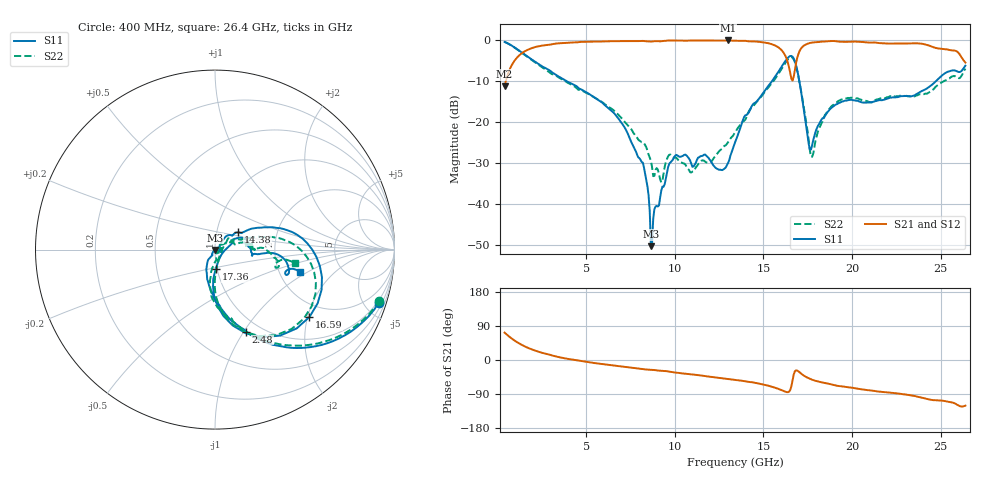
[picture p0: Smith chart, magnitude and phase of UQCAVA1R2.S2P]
!  Part Number  UQCAVA1R2 	Mounting Orientation: Horizontal
!  Description: Ultra Low ESR Microwave capacitors
!  Application: Coupling, Bypass, Tuning, DC Block
!  Filters, Matching
# GHZ S DB R 50
! Freq  |S11|  S11 Ph  |S21|  S21 Ph  |S12|  S12 Ph  |S22|  S22 Ph
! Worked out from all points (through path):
!   401 points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, 400 MHz to 26.4 GHz, reference 50 ohm
!   highest |S21| = 0.00 dB at 13.01 GHz (marker M1); lowest = -11.2 dB at 400 MHz (marker M2)
!   group delay of S21, straight-line fit = 15 ps
!   lowest |S11| = -50.3 dB at 8.655 GHz (marker M3), VSWR 1.01, Z = 49.9 - j0.268 ohm
!   |S11| at or under -10 dB: 3.914 GHz to 15.48 GHz (11.57 GHz wide, 119 % of centre); 17.03 GHz to 24.72 GHz (7.69 GHz wide, 36.8 % of centre)
!   |S22| runs from -34.7 to -0.4 dB; largest |S21 - S12| = 0.0052
!   S11 on the Smith chart (normalised r, x): 400 MHz: 0.83, -6.19; 2.48 GHz: 0.85, -1.02; 14.38 GHz: 1.27, +0.25; 16.59 GHz: 1.59, -2.06; 17.36 GHz: 0.99, -0.22; 26.4 GHz: 2.60, -0.86
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0.4  -0.36 -18.0  -11.17 72.1  -11.20 72.1  -0.37 -17.3
1.18  -2.37 -45.5  -3.83 44.8  -3.85 44.9  -2.40 -44.1
2.48  -6.23 -69.2  -1.29 19.4  -1.31 19.5  -6.46 -70.4
4.755  -12.04 -92.9  -0.35 -3.1  -0.36 -3.0  -12.23 -94.3
7.225  -21.68 -121.0  -0.17 -18.4  -0.16 -18.2  -20.15 -97.3
8.265  -31.10 -125.4  -0.15 -24.5  -0.13 -24.2  -25.11 -79.7
8.655  -50.30 -118.5  -0.26 -25.9  -0.24 -25.6  -29.46 -76.2
9.11  -40.35 1.2  -0.21 -27.9  -0.19 -27.7  -32.67 -37.7
10.085  -27.98 3.5  -0.01 -33.4  -0.01 -33.2  -28.67 5.9
10.995  -30.89 -13.9  -0.01 -37.9  -0.01 -37.8  -32.08 33.7
13.01  -29.93 35.5  0.00 -50.2  -0.01 -50.2  -24.92 33.2
13.4  -24.95 49.0  -0.07 -52.6  -0.05 -52.5  -22.50 29.9
14.375  -15.83 36.5  -0.23 -58.9  -0.21 -58.8  -16.30 21.0
15.935  -7.06 12.6  -1.99 -77.9  -1.97 -77.9  -7.59 5.8
16.585  -3.79 -35.5  -9.38 -68.5  -9.36 -68.6  -4.06 -38.0
16.975  -8.61 -82.9  -3.32 -29.9  -3.30 -29.9  -8.73 -82.2
17.365  -19.30 -87.5  -1.06 -43.6  -1.04 -43.7  -18.51 -86.7
17.755  -25.56 -6.8  -0.51 -52.0  -0.49 -52.1  -28.43 -12.4
19.12  -15.63 23.1  -0.19 -67.6  -0.17 -67.7  -15.20 12.9
22.11  -14.07 1.2  -0.76 -86.0  -0.75 -86.1  -13.71 9.7
23.93  -12.38 -6.2  -0.80 -99.5  -0.78 -99.7  -13.15 -0.6
26.4  -6.17 -14.8  -5.42 -120.5  -5.41 -120.7  -6.87 -9.7
